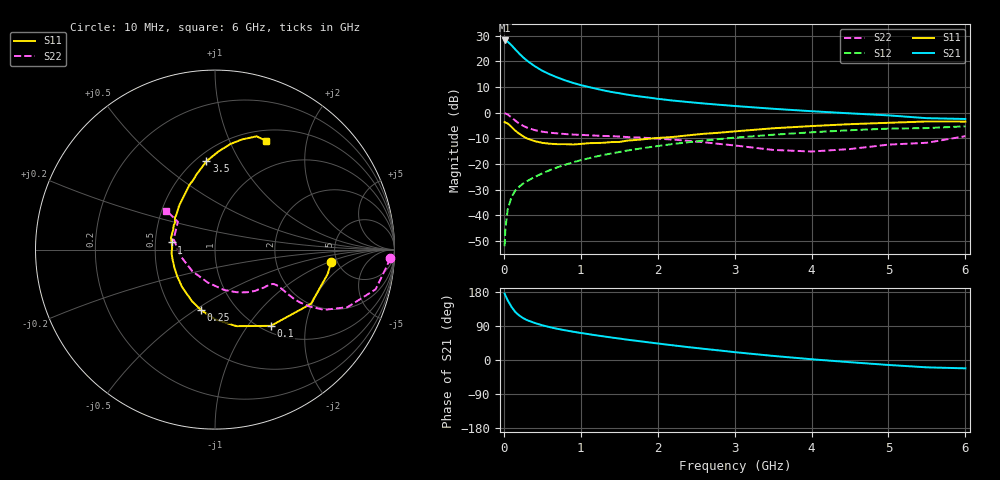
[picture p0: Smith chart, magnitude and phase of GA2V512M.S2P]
! Infineon Technologies  Discrete & RF Semiconductors
! BF775
! Si NPN RF Bipolar Junction Transistor in SOT23
! VCE = 2.5 V  IC = 12 mA
! Common Emitter S-Parameters:  May  1996
# GHz  S  MA  R  50
!  f  S11  S21  S12  S22
! GHz  MAG  ANG  MAG  ANG  MAG  ANG  MAG  ANG
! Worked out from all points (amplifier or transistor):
!   36 points, 10 MHz to 6 GHz, reference 50 ohm
!   highest |S21| = 28.1 dB at 10 MHz (marker M1)
!   |S21| within 3 dB of that: start of sweep to 133.9 MHz
!   unconditionally stable (mu >= 1): 485.5 MHz to 3.396 GHz
!   at 250 MHz: K = 0.75, MSG = 24.6 dB, |S12| = -27.6 dB
!   at 1.4 GHz: K = 1.12, MAG = 9.9 dB, |S12| = -15.9 dB
!   at 6 GHz: K = 0.97, MSG = 1.4 dB, |S12| = -5.3 dB
!   S11 on the Smith chart (normalised r, x): 10 MHz: 4.45, -1.08; 100 MHz: 1.10, -1.30; 250 MHz: 0.69, -0.53; 1 GHz: 0.61, +0.05; 3.5 GHz: 0.56, +0.74; 6 GHz: 0.63, +1.38
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0.01  0.6507 -6.2  25.45 175.2  0.0025 88.7  0.9776 -2.8
0.02  0.6428 -12.1  25.3 170.5  0.0054 85.3  0.96 -5.8
0.05  0.6142 -29.5  24.16 157.6  0.013 77.5  0.9219 -13.9
0.1  0.5265 -53.8  20.47 140.1  0.0229 69.1  0.8045 -23.5
0.15  0.4432 -74.3  16.95 126.4  0.0304 64.4  0.6947 -28.9
0.2  0.3883 -90.0  14.14 117.5  0.036 62.6  0.6133 -31.1
0.25  0.3462 -102.8  11.94 110.6  0.0415 62.0  0.5539 -31.9
0.3  0.3147 -114.1  10.32 105.3  0.0461 62.5  0.5114 -31.9
0.4  0.2779 -131.3  8.053 97.8  0.0557 63.8  0.4571 -31.0
0.5  0.2573 -145.3  6.541 91.6  0.0655 64.8  0.4249 -30.3
0.6  0.2474 -156.2  5.545 86.6  0.0758 65.4  0.4059 -30.0
0.7  0.2426 -166.4  4.808 82.1  0.0863 66.0  0.3932 -30.0
0.8  0.2429 -175.1  4.232 78.3  0.0966 65.6  0.3819 -30.3
1  0.2449 170.6  3.438 71.3  0.1181 65.1  0.3682 -31.7
1.1  0.2537 165.0  3.159 68.3  0.1285 64.4  0.3622 -33.1
1.3  0.2584 154.2  2.704 62.2  0.15 62.8  0.351 -35.6
1.6  0.2844 141.9  2.242 53.7  0.1817 60.2  0.3345 -40.4
2.2  0.3358 122.7  1.715 38.7  0.2445 53.9  0.2977 -52.9
3.5  0.495 95.5  1.188 10.8  0.3705 37.2  0.1876 -102.6
4.5  0.5952 81.6  0.967 -5.8  0.4537 23.7  0.1951 -169.2
5.5  0.6722 69.8  0.779 -19.4  0.4992 9.2  0.2586 143.1
6  0.6691 64.8  0.751 -22.0  0.5409 5.1  0.3474 141.3
